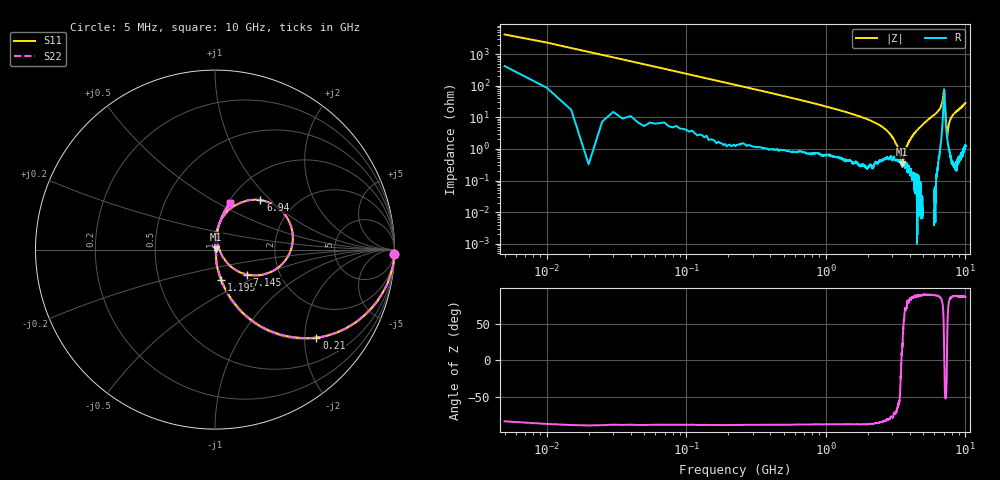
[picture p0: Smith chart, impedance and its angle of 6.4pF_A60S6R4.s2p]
! Amotech Co.,Ltd.
! http://www.amotech.co.kr/
! Part Number: A60S6R4
! These Parameters are Measured in Series Mode Connection
! Operation Temp=25[degC], DC Bias Voltage=0[V]
! Freq. Start=5[MHz] Stop=10[GHz], 2000[Steps]
! Date: Monday, July 13, 2020, 01:55:53
# GHZ S RI R 50.000000
!Freq.(Hz) S11(Real) S11(Imag) S21(Real) S21(Imag) S12(Real) S12(Imag) S22(Real) S22(Imag)
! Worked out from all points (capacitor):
!   2000 points, 5 MHz to 10 GHz, reference 50 ohm
!   read as one part in series: C = 6.67 pF near 55 MHz
!   lowest |Z| = 328 mohm at 3.535 GHz (marker M1)
!   series resonance near 3.478 GHz, so ESL is about 310 pH
!   S11 on the Smith chart (normalised r, x): 5 MHz: 9, -83; 210 MHz: 1.02, -2.28; 1.195 GHz: 1.01, -0.36; 6.94 GHz: 1.36, +0.87; 7.145 GHz: 1.37, -0.40; 10 GHz: 1.02, +0.58
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0.005  0.9971 -0.0236  0.00294 0.0236  0.00294 0.0236  0.9971 -0.0236
0.085  0.8822 -0.313  0.1178 0.313  0.1178 0.313  0.8822 -0.313
0.21  0.5648 -0.4905  0.4352 0.4905  0.4352 0.4905  0.5648 -0.4905
0.53  0.1694 -0.3654  0.8306 0.3654  0.8306 0.3654  0.1694 -0.3654
1.195  0.0358 -0.1709  0.9642 0.1709  0.9642 0.1709  0.0358 -0.1709
1.675  0.0165 -0.1117  0.9835 0.1117  0.9835 0.1117  0.0165 -0.1117
2.855  0.00594 -0.0309  0.9941 0.0309  0.9941 0.0309  0.00594 -0.0309
3.34  0.00433 -0.00632  0.9957 0.00632  0.9957 0.00632  0.00433 -0.00632
3.47  0.00382 -0.000438  0.9962 0.000438  0.9962 0.000438  0.00382 -0.000438
3.535  0.00311 0.00101  0.9969 -0.00101  0.9969 -0.00101  0.00311 0.00101
3.78  0.00374 0.0109  0.9963 -0.0109  0.9963 -0.0109  0.00374 0.0109
3.97  0.00252 0.0179  0.9975 -0.0179  0.9975 -0.0179  0.00252 0.0179
5.005  0.00297 0.0622  0.997 -0.0622  0.997 -0.0622  0.00297 0.0622
6.67  0.0583 0.2005  0.9417 -0.2005  0.9417 -0.2005  0.0583 0.2005
6.94  0.2526 0.2759  0.7474 -0.2759  0.7474 -0.2759  0.2526 0.2759
7.04  0.4332 0.0499  0.5668 -0.0499  0.5668 -0.0499  0.4332 0.0499
7.145  0.1798 -0.1392  0.8202 0.1392  0.8202 0.1392  0.1798 -0.1392
7.345  0.0295 -0.0126  0.9705 0.0126  0.9705 0.0126  0.0295 -0.0126
7.4  0.0224 0.00795  0.9776 -0.00795  0.9776 -0.00795  0.0224 0.00795
7.735  0.0128 0.0759  0.9872 -0.0759  0.9872 -0.0759  0.0128 0.0759
8.335  0.0201 0.1299  0.9799 -0.1299  0.9799 -0.1299  0.0201 0.1299
10  0.0863 0.2604  0.9137 -0.2604  0.9137 -0.2604  0.0863 0.2604
